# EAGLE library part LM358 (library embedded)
OP AMP also LM158; LM258; LM2904 Source: Datasheet
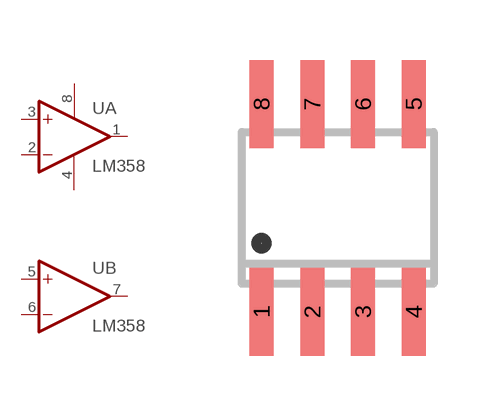
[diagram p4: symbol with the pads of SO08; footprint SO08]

Designator prefix U; gates A=OPAMP B=OPAMP P=PWR+-

## LM358D (DATASHEET: http://www.ti.com/lit/ds/symlink/lm358.pdf; DESCR: Operational Amplifiers - Op Amps Dual Linear - SOIC-8; FARNELL_NO: 1648685; MF: Texas Instruments; MF_PN: LM358D; MOUSER_NO: 595-LM358D; PACKAGE: SOIC-8; PURCHASE: https://de.farnell.com/texas-instruments/lm358dr/op-amp-dual-low-power-soic8-358/dp/1648685; UNIT_PRICE: 0.358)  [SO08]
1  A:OUT  out
2  A:-IN  in
3  A:+IN  in
4  P:V-  pwr
5  B:+IN  in
6  B:-IN  in
7  B:OUT  out
8  P:V+  pwr

## Footprint SO08 (pad centres in mm)
Small Outline Package 8 NS Package M08A
smd 0.6 x 2.2: 1 -1.905,-2.6; 2 -0.635,-2.6; 3 0.635,-2.6; 4 1.905,-2.6; 5 1.905,2.6; 6 0.635,2.6; 7 -0.635,2.6; 8 -1.905,2.6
